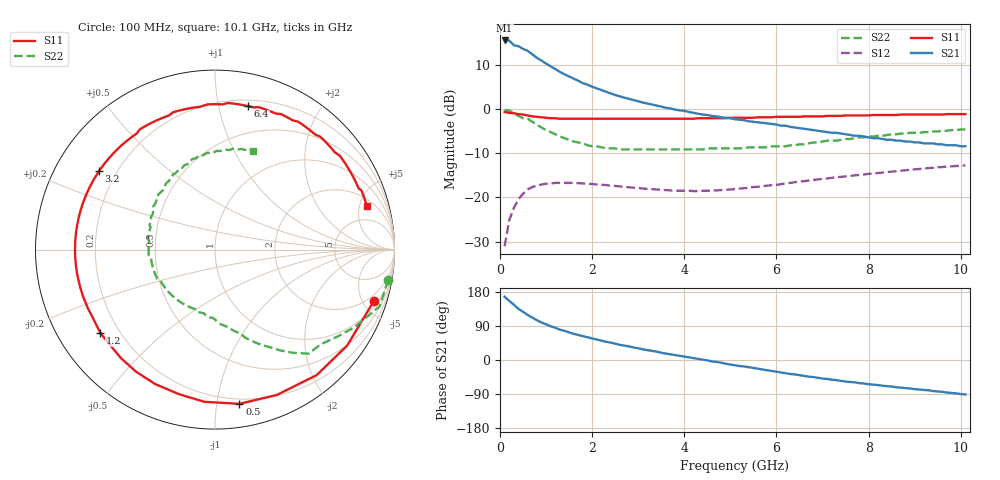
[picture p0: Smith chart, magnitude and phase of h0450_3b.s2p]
!HBFP-0450
!S and NOISE PARAMETERS at Vce=3V  Ic=2mA.  LAST UPDATED  09-04-98
# GHZ S MA R  50
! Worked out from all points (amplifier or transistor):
!   101 points, 100 MHz to 10.1 GHz, reference 50 ohm
!   highest |S21| = 15.6 dB at 100 MHz (marker M1)
!   |S21| within 3 dB of that: start of sweep to 683.5 MHz
!   unconditionally stable (mu >= 1): 3.227 GHz to end of sweep
!   at 1.7 GHz: K = 0.43, MSG = 11.6 dB, |S12| = -16.8 dB
!   at 5.1 GHz: K = 1.46, MAG = 3.9 dB, |S12| = -18.1 dB
!   at 10.1 GHz: K = 1.17, MAG = -0.3 dB, |S12| = -12.7 dB
!   lowest NFmin = 1.31 dB at 1.8 GHz
!   S11 on the Smith chart (normalised r, x): 100 MHz: 1.41, -5.99; 500 MHz: 0.16, -1.16; 1.2 GHz: 0.13, -0.32; 3.2 GHz: 0.13, +0.30; 6.4 GHz: 0.25, +1.23; 10.1 GHz: 2.73, +5.87
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0.1  0.93 -18.0  6.02 167.0  0.028 79.0  0.98 -10.0
0.2  0.91 -36.0  6.01 156.0  0.055 69.0  0.97 -19.0
0.3  0.9 -51.0  5.3 146.0  0.076 59.0  0.89 -29.0
0.4  0.88 -67.0  5.19 135.0  0.095 51.0  0.84 -35.0
0.5  0.87 -81.0  4.83 127.0  0.11 44.0  0.79 -42.0
0.6  0.85 -94.0  4.59 119.0  0.123 38.0  0.78 -48.0
0.8  0.82 -114.0  3.82 105.0  0.136 27.0  0.67 -57.0
0.9  0.81 -123.0  3.56 99.0  0.14 23.0  0.62 -61.0
1  0.8 -131.0  3.29 94.0  0.143 19.0  0.58 -65.0
1.2  0.79 -144.0  2.85 85.0  0.146 12.0  0.52 -71.0
1.3  0.78 -150.0  2.65 80.0  0.146 10.0  0.49 -73.0
1.6  0.78 -164.0  2.22 69.0  0.146 3.0  0.43 -82.0
1.8  0.78 -173.0  1.97 63.0  0.144 -1.0  0.41 -87.0
2.2  0.78 173.0  1.65 51.0  0.139 -7.0  0.37 -98.0
2.5  0.78 164.0  1.45 43.0  0.135 -10.0  0.36 -105.0
3.2  0.78 146.0  1.16 26.0  0.125 -14.0  0.35 -122.0
3.5  0.78 140.0  1.07 19.0  0.122 -15.0  0.35 -130.0
5.1  0.8 104.0  0.77 -14.0  0.124 -14.0  0.36 -168.0
6.4  0.82 77.0  0.62 -38.0  0.149 -19.0  0.39 156.0
6.8  0.83 69.0  0.58 -45.0  0.158 -22.0  0.42 145.0
8.5  0.86 41.0  0.45 -70.0  0.196 -38.0  0.52 104.0
10.1  0.88 16.0  0.38 -91.0  0.231 -60.0  0.59 69.0
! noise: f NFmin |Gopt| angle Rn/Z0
1.8  1.31  0.67  153  0.06
2  1.34  0.65  163  0.05
2.5  1.63  0.71  -176  0.03
3.5  2.14  0.74  -150  0.18
4  2.55  0.75  -134  0.38
5  3.05  0.78  -109  1.08
5.5  3.37  0.8  -97  1.67
7  4.02  0.83  -66  4.12
8  4.46  0.85  -48  6.28
10  4.46  0.9  -17  9.47
